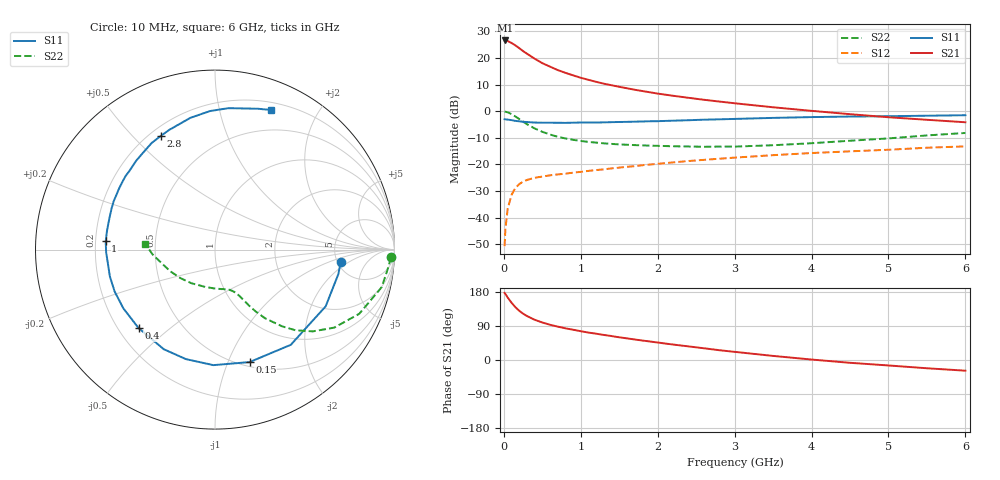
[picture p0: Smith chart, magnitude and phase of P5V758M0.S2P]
! SIEMENS Small Signal Semiconductors
! BFP183
! Si NPN RF Bipolar Junction Transistor in SOT143
! VCE = 0.75 V  IC = 8 mA
! Common Emitter S-Parameters:  March  1996
# GHz  S  MA  R  50
!  f  S11  S21  S12  S22
! GHz  MAG  ANG  MAG  ANG  MAG  ANG  MAG  ANG
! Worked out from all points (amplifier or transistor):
!   36 points, 10 MHz to 6 GHz, reference 50 ohm
!   highest |S21| = 26.6 dB at 20 MHz (marker M1)
!   |S21| within 3 dB of that: start of sweep to 204.9 MHz
!   unconditionally stable (mu >= 1): 1.133 GHz to end of sweep
!   at 250 MHz: K = 0.30, MSG = 24.5 dB, |S12| = -26.5 dB
!   at 1.4 GHz: K = 1.10, MAG = 13.7 dB, |S12| = -21.5 dB
!   at 6 GHz: K = 1.05, MAG = 3.1 dB, |S12| = -13.2 dB
!   S11 on the Smith chart (normalised r, x): 10 MHz: 5.37, -1.44; 150 MHz: 0.55, -1.20; 400 MHz: 0.28, -0.39; 1 GHz: 0.24, +0.04; 2.8 GHz: 0.24, +0.60; 6 GHz: 0.28, +1.44
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0.01  0.7043 -5.5  21.25 177.1  0.0029 86.5  0.9795 -2.5
0.02  0.7007 -11.3  21.3 174.3  0.006 85.5  0.973 -5.2
0.05  0.6928 -27.2  20.8 164.8  0.0146 79.8  0.9521 -12.7
0.1  0.678 -51.5  19.08 151.2  0.0267 66.2  0.8797 -24.0
0.15  0.6556 -72.9  17.21 139.4  0.0361 57.4  0.7939 -33.2
0.2  0.6438 -90.8  15.27 129.9  0.0424 51.0  0.7103 -39.9
0.25  0.6313 -104.9  13.45 122.2  0.0474 46.0  0.6344 -45.1
0.3  0.6241 -117.2  12.04 116.1  0.0509 42.4  0.5684 -48.8
0.4  0.6102 -134.3  9.672 106.2  0.0558 38.0  0.4737 -53.9
0.5  0.6066 -147.4  7.98 99.0  0.059 35.4  0.4094 -56.8
0.6  0.6059 -157.4  6.861 93.0  0.0622 34.3  0.3635 -58.8
0.7  0.6046 -165.7  5.916 88.1  0.0646 34.3  0.3301 -60.1
0.8  0.6017 -172.7  5.253 83.6  0.0668 34.2  0.3068 -61.4
1  0.6107 175.7  4.236 76.0  0.0723 34.3  0.2751 -63.5
1.1  0.6106 170.6  3.877 72.4  0.0754 34.8  0.2642 -64.8
1.5  0.6255 154.4  2.864 59.9  0.0868 35.7  0.2369 -70.6
2.2  0.6618 131.6  1.946 40.8  0.1088 35.0  0.2186 -85.8
2.8  0.7014 115.6  1.515 25.9  0.1276 32.3  0.2157 -102.8
3.5  0.7468 100.6  1.182 10.8  0.1488 28.2  0.2287 -124.9
4.5  0.7915 84.6  0.877 -7.4  0.1756 21.0  0.2778 -154.4
5.5  0.8206 73.0  0.688 -21.8  0.2054 14.3  0.3495 -175.7
6  0.8378 68.2  0.618 -28.2  0.2177 9.9  0.389 175.3
